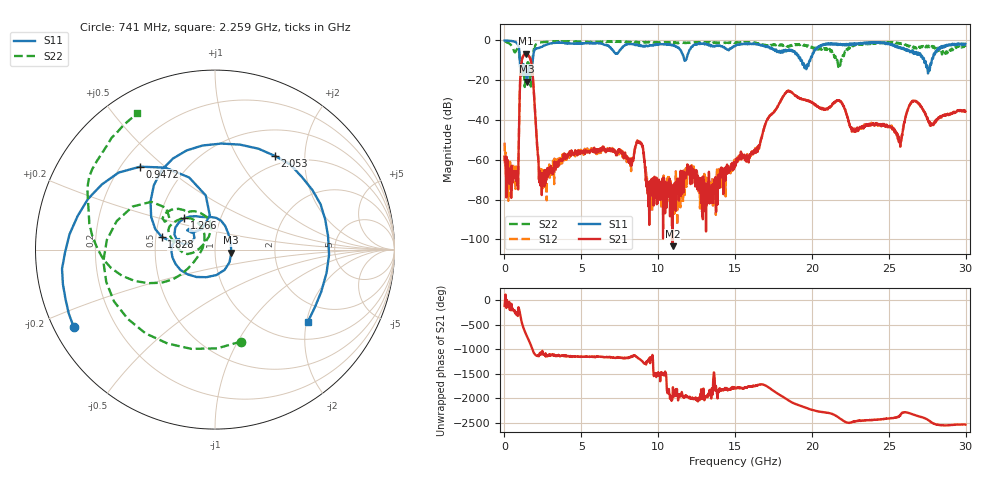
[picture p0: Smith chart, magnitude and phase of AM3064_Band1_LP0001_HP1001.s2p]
# Hz S DB R 50.0
!freq dBS11 angS11 dBS21 angS21 dBS12 angS12 dBS22 angS22
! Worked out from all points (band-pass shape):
!   1600 points, 10 MHz to 29.98 GHz, reference 50 ohm
!   highest |S21| = -6.70 dB at 1.397 GHz (marker M1); lowest = -103.4 dB at 10.94 GHz (marker M2)
!   |S21| within 3 dB of the highest: 1.135 GHz to 1.705 GHz (569.3 MHz wide, 40.1 % of centre)
!   lowest |S11| = -20.7 dB at 1.472 GHz (marker M3), VSWR 1.20, Z = 60 - j2.12 ohm
!   |S11| at or under -10 dB: 1.002 GHz to 1.833 GHz (831.3 MHz wide, 58.7 % of centre); 19.34 GHz to 19.89 GHz (547.8 MHz wide, 2.79 % of centre); 27.3 GHz to 27.79 GHz (496.6 MHz wide, 1.8 % of centre)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
!   |S22| runs from -23.4 to -0.2 dB; largest |S21 - S12| = 0.0055
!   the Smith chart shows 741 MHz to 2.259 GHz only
!   S11 on the Smith chart (normalised r, x): 741 MHz: 0.06, -0.26; 947.2 MHz: 0.28, +0.42; 1.266 GHz: 0.67, +0.25; 1.828 GHz: 0.54, +0.08; 2.053 GHz: 0.86, +1.46; 2.259 GHz: 1.44, -2.04
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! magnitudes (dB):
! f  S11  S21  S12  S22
! 10 MHz  0.0  -58.5  -51.4  -0.2
! 741 MHz  -0.9  -68.9  -64.9  -5.5
! 947.2 MHz  -4.1  -44.1  -44.2  -5.7
! 1.266 GHz  -12.2  -7.3  -7.3  -16.3
! 1.397 GHz  -15.7  -6.7  -6.7  -14.9
! 1.472 GHz  -20.7  -6.9  -6.9  -11.8
! 1.828 GHz  -10.3  -16.4  -16.3  -9.1
! 2.053 GHz  -4.2  -43.6  -43.5  -2.0
! 2.259 GHz  -3.7  -66.9  -68.3  -1.1
! 5.015 GHz  -1.4  -56.0  -56.2  -0.6
! 8.782 GHz  -2.6  -50.9  -51.3  -0.8
! 9.344 GHz  -2.9  -73.7  -76.9  -0.9
! 10 GHz  -2.0  -71.3  -71.6  -0.9
! 10.94 GHz  -2.3  -103.4  -75.6  -1.2
! 15 GHz  -2.7  -61.5  -59.7  -1.3
! 18.34 GHz  -5.5  -26.0  -25.8  -2.8
! 19.99 GHz  -8.3  -31.2  -31.1  -3.3
! 25 GHz  -1.4  -43.2  -43.6  -1.2
! 25.73 GHz  -3.3  -51.4  -49.2  -1.7
! 26.64 GHz  -6.4  -30.4  -30.5  -3.5
! 27.56 GHz  -16.4  -40.6  -40.2  -2.8
! 29.98 GHz  -1.7  -35.8  -35.6  -3.2
